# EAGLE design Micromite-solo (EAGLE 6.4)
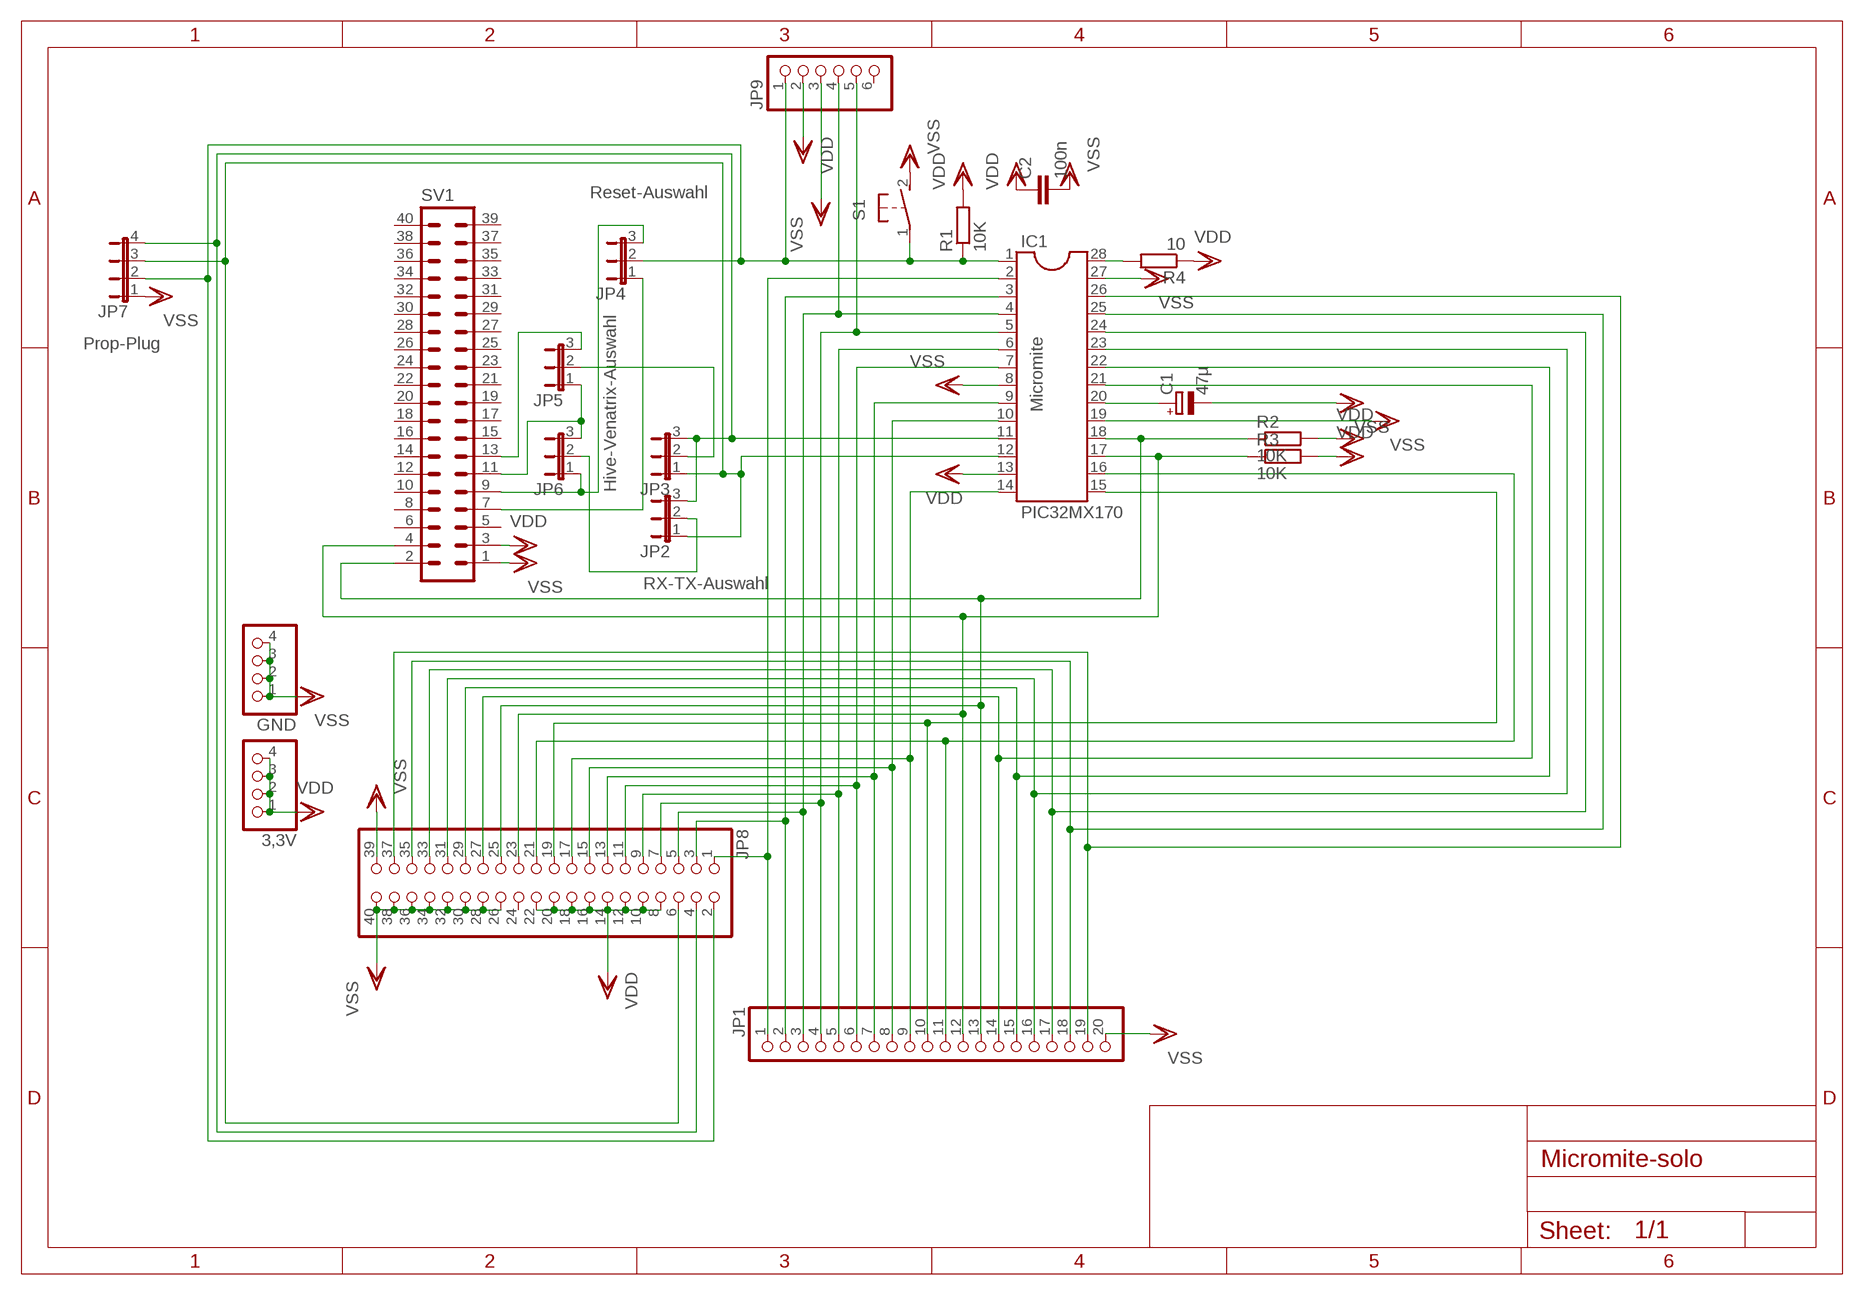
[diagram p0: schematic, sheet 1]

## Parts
3,3V  PINHD-1X4  [1X04]
C1  47µ  CPOL-EUE3.5-8  [E3,5-8]
C2  100n  C-EU025-030X050  [C025-030X050]
GND  PINHD-1X4  [1X04]
IC1  PIC32MX170  DIL28-3  [DIL28-3]
JP1  PINHD-1X20  [1X20]
JP2  JP2E  [JP2]
JP3  JP2E  [JP2]
JP4  JP2E  [JP2]
JP5  JP2E  [JP2]
JP6  JP2E  [JP2]
JP7  JP4E  [JP4]
JP8  PINHD-2X20  [2X20]
JP9  PINHD-1X6  [1X06]
R1  10K  R-EU_0204/7  [0204/7]
R2  10K  R-EU_0204/7  [0204/7]
R3  10K  R-EU_0204/7  [0204/7]
R4  10  R-EU_0204/7  [0204/7]
S1  31-XX  [B3F-31XX]
SV1  ML40L  [ML40L]

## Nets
N$1: IC1.1 JP4.2 JP7.2 JP8.2 JP9.1 R1.1 S1.1(P)
N$2: IC1.18 JP1.13 JP8.25 R2.1 SV1.2
N$3: IC1.17 JP1.12 JP8.23 R3.1 SV1.4
N$4: C1.+ IC1.20
N$5: IC1.28 R4.2
N$6: IC1.2 JP1.1 JP8.1
N$7: IC1.3 JP1.2 JP8.3
N$8: IC1.4 JP1.3 JP8.5 JP9.4
N$9: IC1.5 JP1.4 JP8.7 JP9.5
N$10: IC1.6 JP1.5 JP8.9
N$11: IC1.7 JP1.6 JP8.11
N$12: IC1.26 JP1.19 JP8.37
N$13: IC1.25 JP1.18 JP8.35
N$14: IC1.24 JP1.17 JP8.33
N$15: IC1.23 JP1.16 JP8.31
N$16: IC1.22 JP1.15 JP8.29
N$17: IC1.21 JP1.14 JP8.27
N$18: IC1.16 JP1.11 JP8.21
N$19: IC1.15 JP1.10 JP8.19
N$20: IC1.14 JP1.9 JP8.17
N$21: IC1.9 JP1.7 JP8.13
N$22: IC1.10 JP1.8 JP8.15
N$23: IC1.11 JP2.3 JP3.3 JP7.4 JP8.4
N$24: IC1.12 JP2.1 JP3.1 JP7.3 JP8.6
N$25: JP4.3 JP6.1 SV1.9
N$26: JP5.1 JP6.3 SV1.11
N$27: JP5.3 SV1.13
N$28: JP3.2 JP5.2
N$29: JP4.1 SV1.7
N$30: JP2.2 JP6.2
VDD: 3,3V.1 3,3V.2 3,3V.3 3,3V.4 C2.1 IC1.13 JP8.8 JP8.10 JP8.12 JP8.14 JP8.16 JP8.18 JP8.20 JP8.22 JP9.2 R1.2 R2.2 R3.2 R4.1 SV1.3
VSS: C1.- C2.2 GND.1 GND.2 GND.3 GND.4 IC1.8 IC1.19 IC1.27 JP1.20 JP7.1 JP8.26 JP8.28 JP8.30 JP8.32 JP8.34 JP8.36 JP8.38 JP8.39 JP8.40 JP9.3 S1.2(S) SV1.1
Unconnected: JP8.24 JP9.6 SV1.5 SV1.6 SV1.8 SV1.10 SV1.12 SV1.14 SV1.15 SV1.16 SV1.17 SV1.18 SV1.19 SV1.20 SV1.21 SV1.22 SV1.23 SV1.24 SV1.25 SV1.26 SV1.27 SV1.28 SV1.29 SV1.30 SV1.31 SV1.32 SV1.33 SV1.34 SV1.35 SV1.36 SV1.37 SV1.38 SV1.39 SV1.40

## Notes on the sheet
- Reset-Auswahl
- Prop-Plug
- Micromite
- Hive-Venatrix-Auswahl
- RX-TX-Auswahl

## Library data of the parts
3,3V GND = pinhead:PINHD-1X4: PIN HEADER
C1 = rcl:CPOL-EU: POLARIZED CAPACITOR, European symbol
C2 = rcl:C-EU: CAPACITOR, European symbol
IC1 = ic-package:DIL28: Dual In Line
JP1 = pinhead:PINHD-1X20: PIN HEADER
JP2-JP6 = jumper:JP2E: JUMPER
JP7 = jumper:JP4E: JUMPER
JP8 = pinhead:PINHD-2X20: PIN HEADER
JP9 = pinhead:PINHD-1X6: PIN HEADER
R1-R4 = rcl:R-EU_: RESISTOR, European symbol
S1 = switch-omron:31-XX: OMRON SWITCH; MPN: B3F-3100; OC_FARNELL: 959704; OC_NEWARK: 36M3582
SV1 = con-ml:ML40L: HARTING; OC_FARNELL: unknown; OC_NEWARK: unknown

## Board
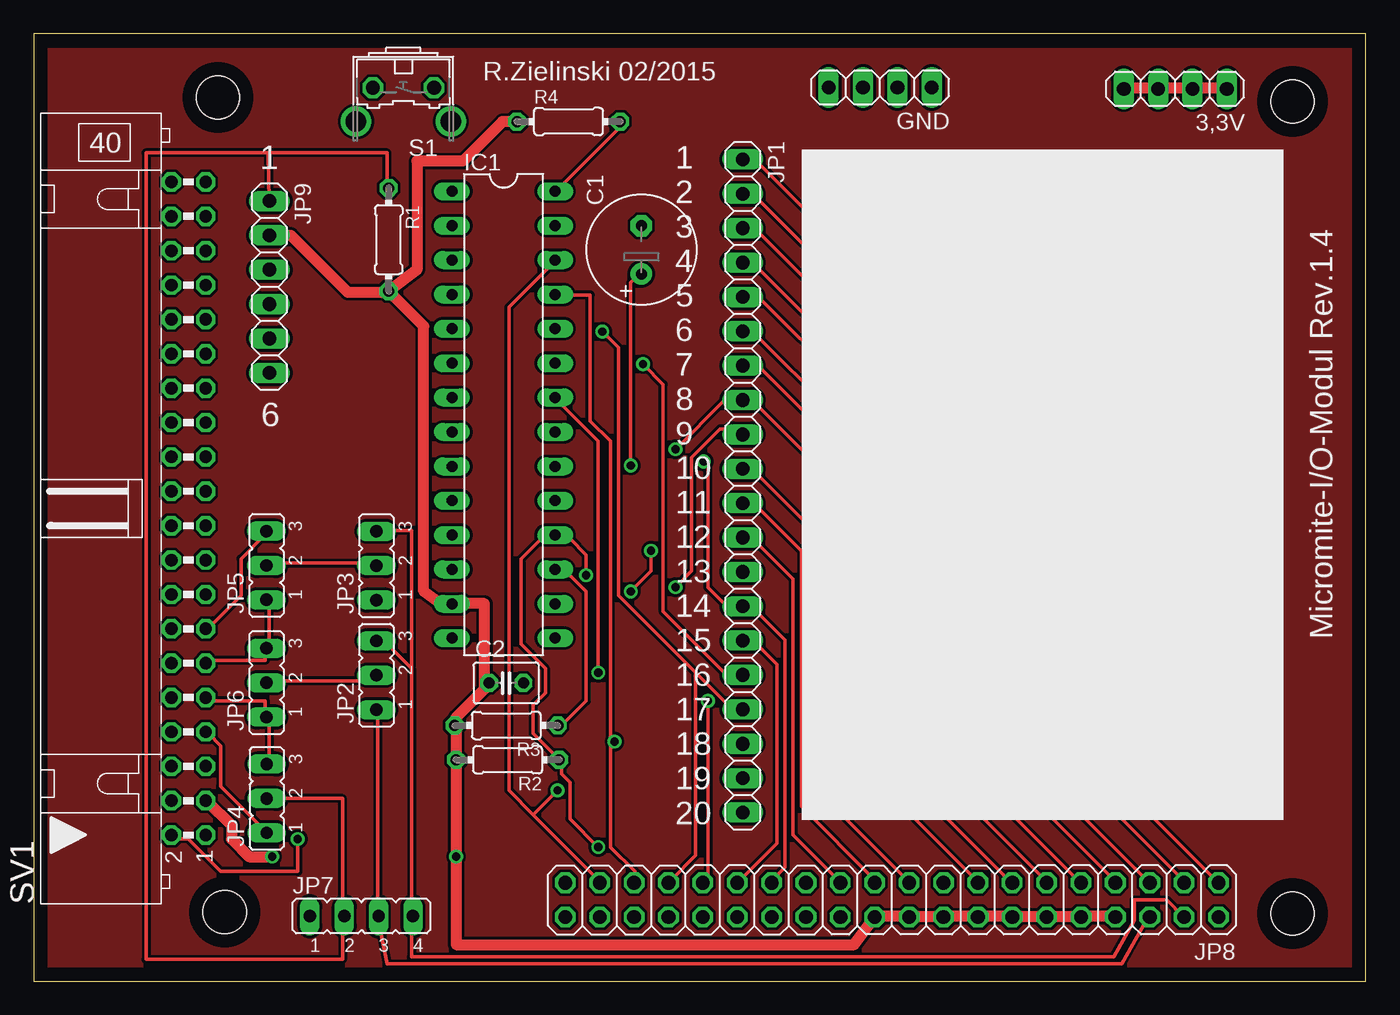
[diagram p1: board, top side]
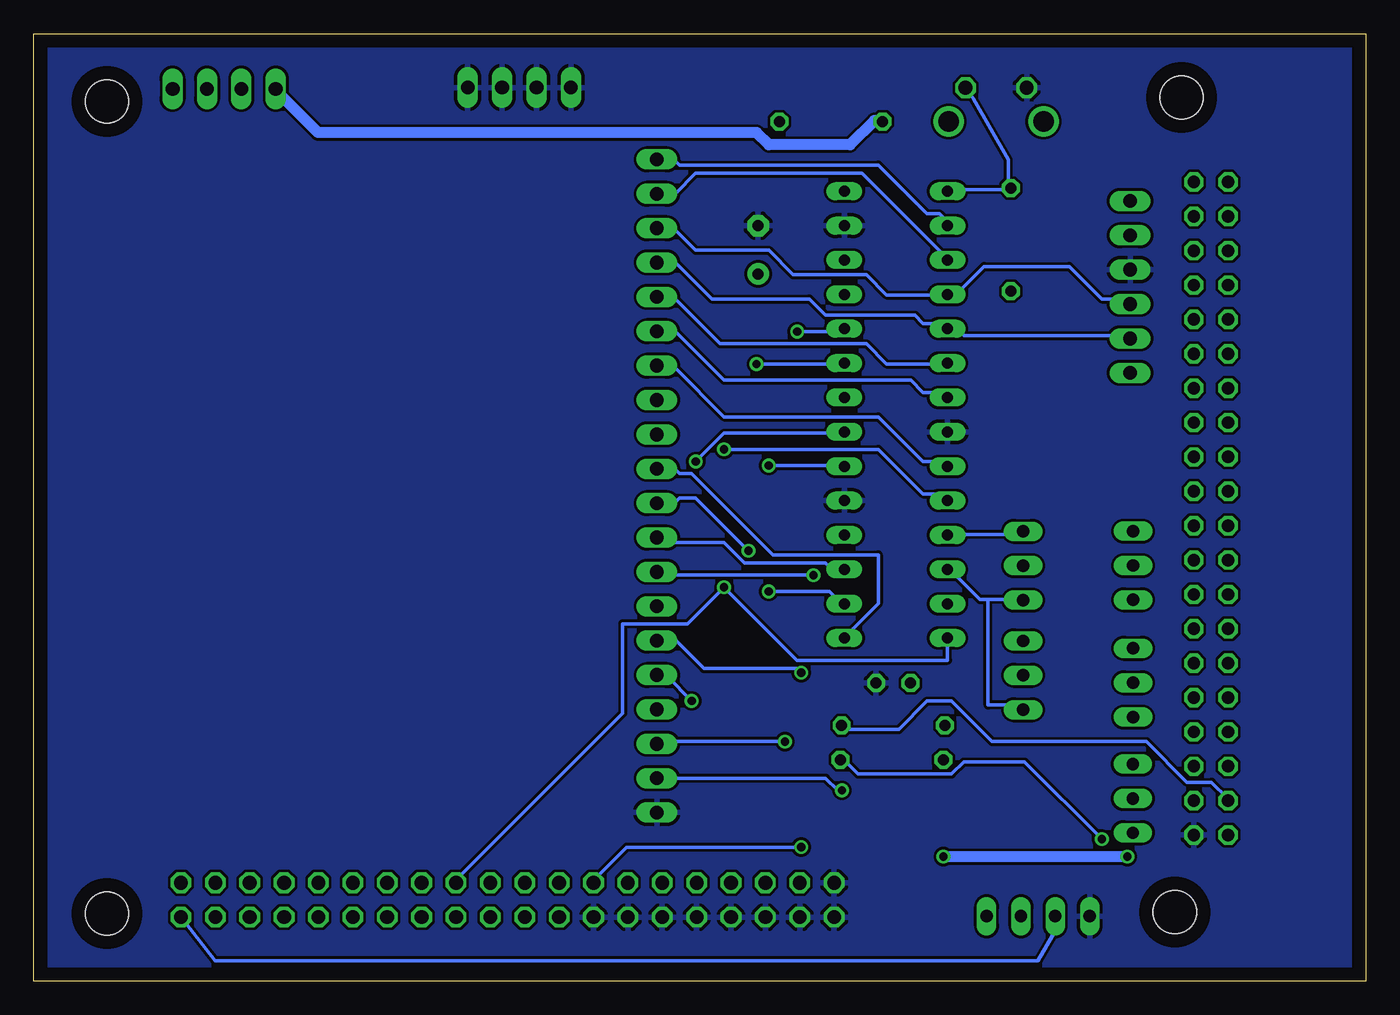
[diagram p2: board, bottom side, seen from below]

Size 98.4 x 70 mm. Coordinates in mm from the lower left corner, seen from the top.
Outline: 0,0 98.4,0 98.4,70 0,70 0,0
Copper layers (1*16): Top 0.035mm / dielectric 1.5mm / Bottom 0.035mm
Design rules "default": minimum track width 10mil, minimum drill 24mil, track to track 8mil, track to pad 8mil, pad to pad 8mil, via to via 8mil, smd to smd 8mil, copper to edge 40mil, drill to drill 8mil, minimum pad ring 10mil, minimum via ring 8mil, stop-mask expansion 4mil, vias tented up to drill 0mil, thermal gap 10mil
Holes 3.2 mm at 93,5 93,65 14.1,5.1 13.6,65.3

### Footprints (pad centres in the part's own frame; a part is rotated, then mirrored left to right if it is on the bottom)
1X04 = drill 1.016 long: 1 -3.81,0; 2 -1.27,0; 3 1.27,0; 4 3.81,0
E3,5-8 = drill 0.813 pad 1.6: + -1.778,0 | drill 0.813 pad 1.6 octagon: - 1.778,0
C025-030X050 = drill 0.813 octagon: 1 -1.27,0; 2 1.27,0
DIL28-3 = drill 0.813 long: 1 -16.51,-3.81; 2 -13.97,-3.81; 3 -11.43,-3.81; 4 -8.89,-3.81; 5 -6.35,-3.81; 6 -3.81,-3.81; 7 -1.27,-3.81; 8 1.27,-3.81; 9 3.81,-3.81; 10 6.35,-3.81; 11 8.89,-3.81; 12 11.43,-3.81; 13 13.97,-3.81; 14 16.51,-3.81; 15 16.51,3.81; 16 13.97,3.81; 17 11.43,3.81; 18 8.89,3.81; 19 6.35,3.81; 20 3.81,3.81; 21 1.27,3.81; 22 -1.27,3.81; 23 -3.81,3.81; 24 -6.35,3.81; 25 -8.89,3.81; 26 -11.43,3.81; 27 -13.97,3.81; 28 -16.51,3.81
1X20 = drill 1.016 long: 1 -24.13,0; 2 -21.59,0; 3 -19.05,0; 4 -16.51,0; 5 -13.97,0; 6 -11.43,0; 7 -8.89,0; 8 -6.35,0; 9 -3.81,0; 10 -1.27,0; 11 1.27,0; 12 3.81,0; 13 6.35,0; 14 8.89,0; 15 11.43,0; 16 13.97,0; 17 16.51,0; 18 19.05,0; 19 21.59,0; 20 24.13,0
JP2 = drill 0.914 long: 1 -2.54,0; 2 0,0; 3 2.54,0
JP4 = drill 0.914 long: 1 -3.81,0; 2 -1.27,0; 3 1.27,0; 4 3.81,0
2X20 = drill 1.016 octagon: 1 -24.13,-1.27; 2 -24.13,1.27; 3 -21.59,-1.27; 4 -21.59,1.27; 5 -19.05,-1.27; 6 -19.05,1.27; 7 -16.51,-1.27; 8 -16.51,1.27; 9 -13.97,-1.27; 10 -13.97,1.27; 11 -11.43,-1.27; 12 -11.43,1.27; 13 -8.89,-1.27; 14 -8.89,1.27; 15 -6.35,-1.27; 16 -6.35,1.27; 17 -3.81,-1.27; 18 -3.81,1.27; 19 -1.27,-1.27; 20 -1.27,1.27; 21 1.27,-1.27; 22 1.27,1.27; 23 3.81,-1.27; 24 3.81,1.27; 25 6.35,-1.27; 26 6.35,1.27; 27 8.89,-1.27; 28 8.89,1.27; 29 11.43,-1.27; 30 11.43,1.27; 31 13.97,-1.27; 32 13.97,1.27; 33 16.51,-1.27; 34 16.51,1.27; 35 19.05,-1.27; 36 19.05,1.27; 37 21.59,-1.27; 38 21.59,1.27; 39 24.13,-1.27; 40 24.13,1.27
1X06 = drill 1.016 long: 1 -6.35,0; 2 -3.81,0; 3 -1.27,0; 4 1.27,0; 5 3.81,0; 6 6.35,0
0204/7 = drill 0.813 octagon: 1 -3.81,0; 2 3.81,0
B3F-31XX = drill 1.016 octagon: 1 -2.261,-1.245; 2 2.261,-1.245 | drill 1.499 pad 2.159: 3 -3.505,1.245; 4 3.505,1.245
ML40L = drill 0.914 octagon: 1 -24.13,-1.27; 2 -24.13,1.27; 3 -21.59,-1.27; 4 -21.59,1.27; 5 -19.05,-1.27; 6 -19.05,1.27; 7 -16.51,-1.27; 8 -16.51,1.27; 9 -13.97,-1.27; 10 -13.97,1.27; 11 -11.43,-1.27; 12 -11.43,1.27; 13 -8.89,-1.27; 14 -8.89,1.27; 15 -6.35,-1.27; 16 -6.35,1.27; 17 -3.81,-1.27; 18 -3.81,1.27; 19 -1.27,-1.27; 20 -1.27,1.27; 21 1.27,-1.27; 22 1.27,1.27; 23 3.81,-1.27; 24 3.81,1.27; 25 6.35,-1.27; 26 6.35,1.27; 27 8.89,-1.27; 28 8.89,1.27; 29 11.43,-1.27; 30 11.43,1.27; 31 13.97,-1.27; 32 13.97,1.27; 33 16.51,-1.27; 34 16.51,1.27; 35 19.05,-1.27; 36 19.05,1.27; 37 21.59,-1.27; 38 21.59,1.27; 39 24.13,-1.27; 40 24.13,1.27

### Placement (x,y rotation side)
3,3V  84.33,65.94 180 top
C1  44.88,54.04 90 top
C2  34.9,22.03 0 top
GND  62.53,66.03 180 top
IC1  34.7,41.85 270 top
JP1  52.37,36.59 270 top
JP2  25.3,22.6 90 top
JP3  25.3,30.7 90 top
JP4  17.2,13.5 90 top
JP5  17.18,30.71 90 top
JP6  17.18,22.05 90 top
JP7  24.2,4.8 0 top
JP8  63.4,6 180 top
JP9  17.4,51.3 270 top
R1  26.22,54.79 270 top
R2  35.01,16.36 180 top
R3  34.91,18.89 180 top
R4  39.51,63.52 0 top
S1  27.3,64.77 180 top
SV1  11.43,34.92 90 top

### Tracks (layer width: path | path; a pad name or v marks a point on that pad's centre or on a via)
N$1
  Top 0.254: 17.3,61.2 26.1,61.2 26.1,58.5 R1.1 | JP4.2 22.8,13.5 22.8,4.8 | 22.8,4.8 22.8,1.6 8.3,1.6 8.3,61.2 17.3,61.2 | 22.8,4.8 JP7.2 | 17.3,61.2 JP9.1
  Bottom 0.254: IC1.1 30.6,58.5 26.4,58.5 R1.1 26.4,58.8 26.4,60.7 29,65.2 S1.1 | JP8.2 85,1.5 24.2,1.5 22.9,3.8 22.9,4.8 JP7.2
N$2  (via drill 0.61)
  Top 0.254: v41.7,9.9 39.6,12 39.6,14.7 39,15.3 39,16.2 R2.1 38.7,16.5 36.9,18.3 36.9,20.4 37.8,21.3 37.8,23.1 36,24.9 36,31.2 37.5,32.7 38.4,32.7 IC1.18 38.7,32.7 39.6,32.7 40.8,31.5 v40.8,30 | v19.5,10.5 19.5,8.1 13.8,8.1 11.4,10.5 10.2,10.5 SV1.2
  Bottom 0.254: v41.7,9.9 54.6,9.9 57,7.5 JP8.25 | v40.8,30 52.2,30 JP1.13 | v19.5,10.5 25.2,16.2 29.7,16.2 30.6,15.3 37.5,15.3 38.4,16.2 38.7,16.2 R2.1
N$3
  Top 0.254: R3.1 39,18.9 40.8,20.7 40.8,28.8 39.3,30.3 38.7,30.3 IC1.17 | JP8.23 59.4,7.5 56.1,10.8 56.1,29.7 53.1,32.7 52.5,32.7 JP1.12
  Bottom 0.254: JP1.12 52.2,32.7 51.9,32.4 47.4,32.4 45.9,30.9 39.9,30.9 39.6,30.6 38.7,30.6 IC1.17 | SV1.4 10.2,13.5 11.4,14.7 13.2,14.7 16.2,17.7 27.6,17.7 30.6,20.7 32.4,20.7 34.5,18.6 38.7,18.6 R3.1
N$4  (via drill 0.61)
  Top 0.254: v44.1,38.1 44.1,51.6 44.7,52.2 C1.+
  Bottom 0.254: v44.1,38.1 38.7,38.1 IC1.20
N$5
  Top 0.254: IC1.28 38.7,58.5 43.2,63 43.2,63.3 R4.2
N$6
  Top 0.254: JP8.1 62.1,32.7 62.1,51.9 53.4,60.6 52.5,60.6 JP1.1
  Bottom 0.254: IC1.2 30.9,56.1 31.5,56.7 32.4,56.7 36,60.3 50.7,60.3 51,60.6 52.2,60.6 JP1.1
N$7
  Top 0.254: JP8.3 84.9,7.5 61.5,30.9 61.5,49.8 53.4,57.9 52.5,57.9 JP1.2
  Bottom 0.254: IC1.3 30.9,53.4 37.2,59.7 49.5,59.7 51,58.2 52.2,58.2 JP1.2
N$8
  Top 0.254: JP8.5 82.2,7.5 60.9,28.8 60.9,48 53.4,55.5 52.5,55.5 JP1.3
  Bottom 0.254: JP1.3 52.2,55.5 51,55.5 49.5,54 44.1,54 42.3,52.2 36.9,52.2 35.4,50.7 30.9,50.7 IC1.4 30.6,51 30,51 28.2,52.8 21.9,52.8 19.5,50.4 17.7,50.4 17.4,50.1 JP9.4
N$9
  Top 0.254: JP1.4 53.1,53.1 60.3,45.9 60.3,27 79.8,7.5 JP8.7
  Bottom 0.254: JP1.4 51,53.1 48.3,50.4 41.1,50.4 39.9,49.2 33.3,49.2 32.7,48.6 31.2,48.6 30.9,48.3 IC1.5 30.6,48 30,48 29.7,47.7 17.4,47.7 JP9.5
N$10
  Top 0.254: JP8.9 77.1,7.5 59.7,24.9 59.7,44.4 53.7,50.4 52.5,50.4 JP1.5
  Bottom 0.254: IC1.6 30.9,45.6 35.4,45.6 36.9,47.1 47.7,47.1 51,50.4 52.2,50.4 JP1.5
N$11
  Top 0.254: JP8.11 74.7,7.5 59.1,23.1 59.1,42 53.1,48 52.5,48 JP1.6
  Bottom 0.254: IC1.7 30.9,43.2 31.2,43.5 32.7,43.5 33.6,44.4 47.4,44.4 51,48 52.2,48 JP1.6
N$12  (via drill 0.61)
  Top 0.254: 36.9,12.3 41.7,7.5 JP8.37 | 36.9,12.3 35.1,14.1 35.1,49.8 38.4,53.1 IC1.26 | 36.9,12.3 v38.7,14.1
  Bottom 0.254: JP1.19 39.9,15 39,14.1 v38.7,14.1
N$13  (via drill 0.61)
  Top 0.254: 42.6,17.7 42.6,9.9 44.4,8.1 44.4,7.5 JP8.35 | 42.6,17.7 42.6,39.9 41.1,41.4 41.1,50.7 38.7,50.7 IC1.25 | 42.6,17.7 v42.9,17.7
  Bottom 0.254: v42.9,17.7 52.2,17.7 JP1.18
N$14  (via drill 0.61)
  Top 0.254: v42,48 43.2,46.8 43.2,28.5 48.9,22.8 | 48.9,22.8 51.6,20.1 52.2,20.1 JP1.17 | 48.9,22.8 48.9,9.3 47.1,7.5 JP8.33
  Bottom 0.254: v42,48 38.7,48 IC1.24
N$15  (via drill 0.61)
  Top 0.254: v45,45.6 46.5,44.1 46.5,27.3 51,22.8 52.2,22.8 JP1.16 | v49.8,20.7 49.8,7.8 49.5,7.5 JP8.31
  Bottom 0.254: v45,45.6 38.7,45.6 IC1.23 | v49.8,20.7 51.6,22.5 52.2,22.5 JP1.16
N$16  (via drill 0.61)
  Top 0.254: v41.7,22.8 41.7,39.9 38.7,42.9 IC1.22 | JP8.29 54.9,10.2 54.9,23.4 53.4,24.9 52.5,24.9 JP1.15
  Bottom 0.254: v41.7,22.8 42,23.1 48.9,23.1 51,25.2 52.2,25.2 JP1.15
N$17  (via drill 0.61)
  Top 0.254: v49.5,38.4 49.8,38.1 49.8,29.1 51,27.9 52.2,27.9 JP1.14 52.5,27.6 53.1,27.6 55.5,25.2 55.5,8.4 54.6,7.5 JP8.27
  Bottom 0.254: v49.5,38.4 47.4,40.5 38.7,40.5 IC1.21
N$18  (via drill 0.61)
  Top 0.254: v44.1,28.8 45.6,30.3 v45.6,31.8 | JP8.21 62.1,7.5 56.7,12.9 56.7,31.8 53.4,35.1 52.5,35.1 JP1.11
  Bottom 0.254: v44.1,28.8 39.6,28.8 38.7,27.9 IC1.16 | v45.6,31.8 49.5,35.7 50.7,35.7 51,35.4 52.2,35.4 JP1.11
N$19
  Top 0.254: JP8.19 64.5,7.5 57.3,14.7 57.3,33.6 53.1,37.8 52.5,37.8 JP1.10
  Bottom 0.254: IC1.15 38.4,25.5 36,27.9 36,31.5 43.8,31.5 49.8,37.5 50.7,37.5 51,37.8 52.2,37.8 JP1.10
N$20  (via drill 0.61)
  Top 0.254: v47.4,29.1 48.6,30.3 48.6,38.7 50.7,40.8 52.2,40.8 52.2,40.5 JP1.9
  Bottom 0.254: IC1.14 30.9,25.2 30.9,23.7 42,23.7 v47.4,29.1 50.1,26.4 54.9,26.4 54.9,19.8 67.2,7.5 JP8.17
N$21
  Top 0.254: JP8.13 72,7.5 58.5,21 58.5,40.5 53.7,45.3 52.5,45.3 JP1.7
  Bottom 0.254: IC1.9 30.9,38.1 31.2,38.4 32.7,38.4 36,41.7 47.4,41.7 51,45.3 52.2,45.3 JP1.7
N$22  (via drill 0.61)
  Top 0.254: v47.4,39.3 51,42.9 52.2,42.9 JP1.8 52.5,42.9 53.1,42.9 57.9,38.1 57.9,19.2 69.6,7.5 JP8.15
  Bottom 0.254: v47.4,39.3 36,39.3 32.7,36 31.2,36 30.9,35.7 IC1.10
N$23
  Top 0.254: 27.9,4.8 JP7.4 | 27.9,23.1 27.9,4.8 | 27.9,23.1 26.1,24.9 25.5,24.9 JP2.3 | 27.9,4.8 27.9,1.8 79.8,1.8 81.3,4.5 81.3,6 83.7,6 84.9,4.8 JP8.4 | 27.9,23.1 27.9,33.3 25.5,33.3 JP3.3
  Bottom 0.254: IC1.11 30.6,33 25.5,33 JP3.3
N$24
  Top 0.254: 25.4,4.7 25.4,19.8 JP2.1 | 25.4,4.7 26.1,1.3 80.4,1.3 82.2,4.5 JP8.6 | 25.4,4.7 JP7.3
  Bottom 0.254: 27.9,28.2 25.5,28.2 JP3.1 | 27.9,28.2 28.5,28.2 30.6,30.3 IC1.12 | 27.9,28.2 27.9,20.4 25.8,20.4 25.5,20.1 JP2.1
N$25
  Top 0.254: SV1.9 12.9,20.7 17.1,20.7 17.1,19.8 JP6.1 17.4,19.5 17.4,16.2 JP4.3
N$26
  Top 0.254: JP5.1 17.4,27.9 17.4,24.6 JP6.3 17.1,24.3 17.1,23.7 12.9,23.7 SV1.11
N$27
  Top 0.254: SV1.13 12.9,26.1 15.3,28.5 15.3,31.2 17.1,33 JP5.3
N$28
  Top 0.254: JP3.2 25.2,30.9 17.4,30.9 JP5.2
N$29
  Top 0.254: JP4.1 17.1,11.1 13.8,14.4 13.8,17.4 12.9,18.3 SV1.7
N$30
  Top 0.254: JP6.2 17.4,22.2 25.2,22.2 25.2,22.5 JP2.2
N$31
  pour Top: 0.9,69 97.6,68.9 97.6,0.7 0.7,0.8
VDD  (via drill 0.61)
  Top 0.254: 82.8,66 3,3V.3 83.1,66 | 85.8,66 3,3V.2 85.5,66 | 64.5,4.8 JP8.20 64.8,4.8 | 67.2,4.8 JP8.18 67.5,4.8 | 77.4,4.8 JP8.10 77.1,4.8 | 79.8,4.8 JP8.8 | 69.9,4.8 JP8.16 69.6,4.8 | 72,4.8 JP8.14 72.3,4.8 | 74.7,4.8 JP8.12 75,4.8 | 33.3,21.6 33.6,21.9 C2.1 | 31.2,18.9 R3.2 31.2,18.6 | 31.2,16.5 R2.2 31.2,16.2
  Top 0.813: 82.8,66 80.7,66 3,3V.4 | 85.8,66 87.9,66 3,3V.1 | 85.5,66 83.1,66 | 64.5,4.8 62.4,4.8 JP8.22 62.1,4.7 60.6,2.7 31.2,2.7 v31.2,9.2 31.2,16.2 | 64.8,4.8 67.2,4.8 | 79.8,4.8 77.4,4.8 | 72,4.8 69.9,4.8 | 72.3,4.8 74.7,4.8 | 75,4.8 77.1,4.8 | 69.6,4.8 67.5,4.8 | 33.3,21.6 31.2,19.5 31.2,18.9 | 30.9,27.9 33.3,27.9 33.3,21.6 | 30.9,27.9 IC1.13 | 33.3,21.6 C2.1 | 31.2,18.6 31.2,16.5 | SV1.3 12.77,13.34 14.6,11.5 14.6,10.5 15.9,9.2 v17.6,9.2 | 30.9,27.9 30,27.9 28.8,28.8 28.8,48.4 R1.2 | JP9.2 18.99,55.11 23.2,50.9 26.14,50.9 R1.2 | R1.2 26.22,50.92 26.2,50.9 | R4.1 34.62,63.52 31.7,60.6 28.3,60.6 28.3,52.56 R1.2
  Bottom 0.254: 80.4,65.7 3,3V.4 | 35.7,63.6 R4.1
  Bottom 0.813: 80.4,65.7 77.4,62.7 45,62.7 44.1,61.8 38.1,61.8 36.3,63.6 35.7,63.6 | v17.6,9.2 v31.2,9.2
VSS
  pour Bottom: 0.64,69.22 97.47,69.42 97.78,0.83 0.94,0.64

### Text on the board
tNames: R.Zielinski 02/2015 | 1 | Micromite-I/O-Modul Rev.1.4 | 6 | 1 / 2 / 3 / 4 / 5 / 6 / 7 / 8 / 9 / 10 / 11 / 12 / 13 / 14 / 15 / 16 / 17 / 18 / 19 / 20
tDocu: 1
